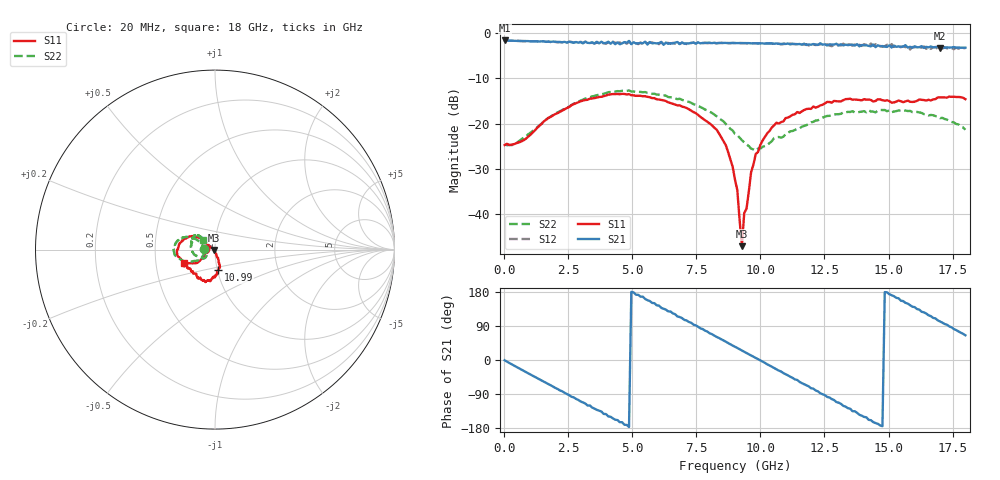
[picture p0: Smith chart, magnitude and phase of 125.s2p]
!Agilent Technologies,N5230A,US43500223,A.07.50.48
!Agilent N5230A: A.07.50.48
!Date: Monday, January 18, 2016 15:46:10
!Correction: S11(Full 2 Port(1,2))
!S21(Full 2 Port(1,2))
!S12(Full 2 Port(1,2))
!S22(Full 2 Port(1,2))
!S2P File: Measurements: S11, S21, S12, S22:
# Hz S  dB  R 50
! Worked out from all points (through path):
!   201 points, 20 MHz to 18 GHz, reference 50 ohm
!   highest |S21| = -1.61 dB at 20 MHz (marker M1); lowest = -3.2 dB at 17.01 GHz (marker M2)
!   group delay of S21, straight-line fit = 101 ps
!   lowest |S11| = -47.1 dB at 9.28 GHz (marker M3), VSWR 1.01, Z = 49.6 - j0.131 ohm
!   |S11| at or under -10 dB: start of sweep to end of sweep
!   |S22| runs from -25.9 to -12.7 dB; largest |S21 - S12| = 0.078
!   S11 on the Smith chart (normalised r, x): 20 MHz: 0.89, +0.00; 10.99 GHz: 1.01, -0.23; 18 GHz: 0.70, -0.11
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2e7  -24.73 179.2  -1.61 -0.8  -1.60 -0.9  -24.59 179.2
1.5483e9  -19.52 -143.5  -1.80 -57.4  -1.79 -57.8  -19.50 -147.4
3.0766e9  -14.90 -155.7  -2.25 -112.2  -2.14 -112.7  -14.70 -159.2
3.7958e9  -14.06 -165.3  -1.88 -135.8  -2.14 -136.2  -13.53 -167.7
4.8746e9  -13.48 -179.6  -1.69 -176.8  -1.91 -175.9  -12.67 178.3
6.0433e9  -14.67 162.5  -2.19 143.6  -2.43 142.2  -13.60 164.5
6.7625e9  -15.96 152.7  -1.94 114.8  -2.02 114.8  -14.59 158.2
7.5716e9  -18.09 146.0  -2.03 87.7  -2.03 87.2  -16.10 153.0
8.6504e9  -24.76 143.2  -2.15 48.2  -2.16 47.2  -20.08 153.0
9.01e9  -32.42 153.0  -2.17 35.0  -2.20 33.6  -22.28 157.3
9.0999e9  -34.69 151.7  -2.18 31.7  -2.20 30.7  -22.54 161.3
9.2797e9  -47.11 -162.5  -2.18 25.2  -2.20 23.9  -23.67 166.2
9.3696e9  -39.78 -112.2  -2.18 21.7  -2.20 20.7  -24.14 167.2
9.8191e9  -26.73 -73.7  -2.22 5.1  -2.22 4.1  -25.94 -165.7
1.09878e10  -18.77 -81.6  -2.38 -37.8  -2.28 -39.0  -22.31 -141.0
1.20666e10  -16.21 -90.2  -2.39 -75.7  -2.50 -78.6  -19.61 -159.4
1.35949e10  -14.72 -105.7  -2.52 -135.1  -2.76 -133.5  -17.24 171.7
1.43141e10  -14.78 -115.0  -2.90 -158.8  -2.28 -162.4  -17.34 160.3
1.50333e10  -15.02 -126.0  -2.67 173.6  -3.04 173.6  -17.06 150.3
1.61121e10  -14.96 -144.2  -3.12 134.4  -2.96 134.2  -17.41 142.1
1.70111e10  -14.22 -151.1  -3.25 101.6  -3.01 98.7  -18.79 140.2
1.8e10  -14.60 -156.4  -3.20 65.2  -3.30 63.6  -21.34 142.2
